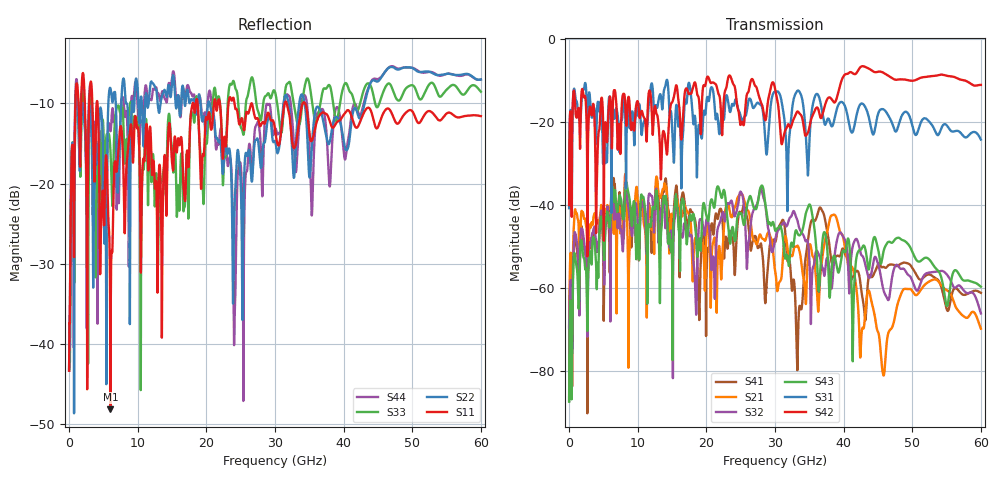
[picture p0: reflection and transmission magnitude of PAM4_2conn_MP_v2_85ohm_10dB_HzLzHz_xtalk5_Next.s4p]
! Info: Touchstone file created by Circ.  Input file=FAB50GbE_2conn_Midplane_Examax_Topo2_v2_85ohm_10dB_HzLzHz.circ
# Hz S RI R 50
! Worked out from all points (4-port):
!   6000 points, 10 MHz to 60 GHz, reference 50 ohm
!   strongest paths, dB at 10 MHz, 15.01 GHz, 30.01 GHz, 45.01 GHz, 60 GHz:
!     S42: -40.1, -15.4, -12.0, -8.0, -11.2
!     S31: -40.9, -21.6, -12.8, -18.2, -24.3
!     S43: -87.5, -51.0, -46.1, -50.6, -59.8
!     S32: -69.7, -53.5, -48.4, -54.2, -66.2
!     S21: -69.3, -45.1, -55.7, -70.7, -69.9
!     S41: -87.2, -43.0, -49.0, -54.4, -61.3
!   lowest |S11| = -48.2 dB at 6.03 GHz (marker M1), VSWR 1.01, Z = 49.9 + j0.386 ohm
!   |S11| at or under -10 dB: 4.142 GHz to 18 GHz (13.86 GHz wide, 125 % of centre); 26.63 GHz to 31.41 GHz (4.774 GHz wide, 16.5 % of centre); 34.4 GHz to end of sweep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
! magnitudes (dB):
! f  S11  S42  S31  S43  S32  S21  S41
! 10 MHz  -43.4  -40.1  -40.9  -87.5  -69.7  -69.3  -87.2
! 2.03 GHz  -6.2  -12.8  -12.4  -52.0  -46.9  -41.9  -48.1
! 6.03 GHz  -48.2  -14.5  -17.5  -43.8  -61.6  -41.6  -45.1
! 24.12 GHz  -10.2  -11.5  -15.4  -48.7  -42.8  -40.8  -56.5
! 38.72 GHz  -12.7  -15.4  -19.0  -52.6  -51.8  -42.5  -52.9
! 45.77 GHz  -11.2  -8.2  -17.0  -51.6  -60.3  -80.9  -55.0
! 60 GHz  -11.6  -11.2  -24.3  -59.8  -66.2  -69.9  -61.3
